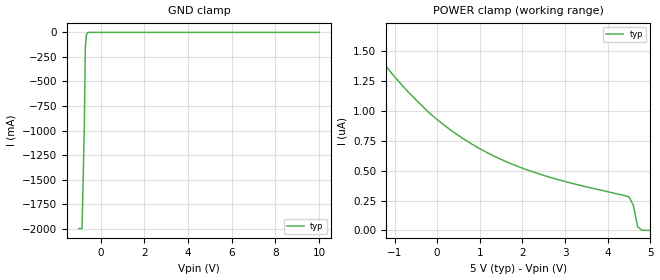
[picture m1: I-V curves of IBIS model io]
|Texas Instruments Incorporated
|2-Channel Ultra-Low Clamp Voltage ESD Solution With Series-Resistor Isolation
| Marketing part#   Digital Voltage Range   Package-type   #pins
| TPD2S017DBVR   0V-5V   SOT-23   6
[IBIS Ver]   4.1
[File name]   tpd2s017.ibs
[File Rev]   1.0
[Date]   10/28/2016
[Source]
| Texas Instruments Incorporated.
| Analog-eLab Design Center, HPA
| 12500 TI Blvd
| Dallas, TX -75243
[Notes]   Revision History:
| Rev 1.0: 10/28/2016
| - Initial version of the model
| - Model generated from bench data
| - Only nominal corner modeled.
| - C_comp although listed in numerical order of value are
|   obtained from varying PVT conditions. For PVT conditions for
|   each specific value refer the buffer description under
|   respective [Model]. IBIS model user is responsible for using
|   appropriate C_comp to simulate for Signal Integrity.
[Disclaimer]
| This model is designed as an aid for customers of Texas Instruments.
| TI and its licensors and suppliers make no warranties, either expressed
| or implied, with respect to this  model, including the warranties of
| merchantability or fitness for a particular purpose. The model is
| provided solely on an "as is" basis. The entire risk as to its quality
| and performance is with the customer.
[Copyright]
(C) Copyright 2016 Texas Instruments Incorporated.All rights reserved.
|   TPD2S017DBV
[Component]   TPD2S017DBV
[Manufacturer]   TI
[Package]   |6 SOT-23 - DBV package
|   typ   min   max
R_pkg   0.0792   0.0646   0.0861
L_pkg   1.8700n   1.5304n   2.0081n
C_pkg   0.2499p   0.2175p   0.2699p
[Pin]  signal_name model_name   R_pin   L_pin   C_pin
1   Ch1_Out   io   na   na   na
2   GND   gnd   na   na   na
3   Ch1_In   io   na   na   na
4   Ch2_In   io   na   na   na
5   VCC   power   na   na   na
6   Ch2_Out   io   na   na   na
| Models and submodels in the file (1): io (Terminator)
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|   io Model
[Model]   io
Model_type   Terminator
|   typ   min   max
C_comp   1.000e-200   1.000e-200   1.000e-200
| Where nom  PVT is Nominal Process, 5V,   25C
|   Fast PVT is Strong Process,  5.25V, -40C
|   Slow PVT is Weak Process,   4.75V, 125C
[Voltage Range]   5   4.75   5.25
|Ambient Temperature   25   125   -40
|Junction Temperature
[Temperature Range]   25   125   -40
[Power Clamp Reference]   5   4.75   5.25
[GND Clamp Reference]   0   0   0
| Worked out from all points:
|   GND clamp passes 1 mA (typ) near -0.56 V on its own axis
[GND Clamp]
|   Voltage   I(typ)   I(min)   I(max)
-1V       -1.999A    NA         NA
-850mV    -1.999A    NA         NA
-750mV    -993mA     NA         NA
-700mV    -154.9mA   NA         NA
-650mV    -23.49mA   NA         NA
-600mV    -3.513mA   NA         NA
10V       0A         NA         NA
[Power Clamp]
|   Voltage   I(typ)   I(min)   I(max)
-5V       31.98uA    NA         NA
-1.8V     1.69uA     NA         NA
-1.3V     1.421uA    NA         NA
-700mV    1.167uA    NA         NA
-200mV    988.3nA    NA         NA
400mV     819.2nA    NA         NA
1.2V      645.6nA    NA         NA
2V        521.1nA    NA         NA
4.5V      279.9nA    NA         NA
4.6V      209nA      NA         NA
4.7V      31.64nA    NA         NA
5V        80pA       NA         NA
